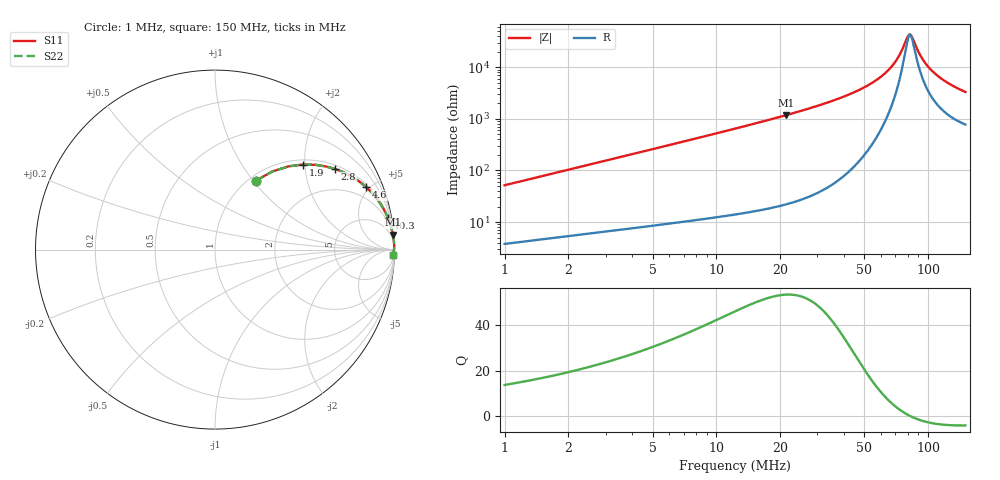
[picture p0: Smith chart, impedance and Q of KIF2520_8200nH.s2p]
!version-2
!date-12.2020
!Series
# MHz S RI R 50
!Freq ReS11 ImS11 ReS21 ImS21 ReS12 ImS12 ReS22 ImS22
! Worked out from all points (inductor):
!   498 points, 1 MHz to 150 MHz, reference 50 ohm
!   read as one part in series: L = 8.2 uH near 1.6 MHz
!   highest Q = 53.6 at 21.4 MHz (marker M1), where L = 8.8 uH
!   self-resonance near 82 MHz
!   S11 on the Smith chart (normalised r, x): 1 MHz: 1.08, +1.03; 1.9 MHz: 1.10, +1.96; 2.8 MHz: 1.13, +2.89; 4.6 MHz: 1.16, +4.75; 10.3 MHz: 1, +11; 150 MHz: 17, -65
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1  0.2269 0.3839  0.7731 -0.3839  0.7731 -0.3839  0.2269 0.3839
1.9  0.4908 0.4741  0.5092 -0.4741  0.5092 -0.4741  0.4908 0.4741
2.8  0.6694 0.4491  0.3306 -0.4491  0.3306 -0.4491  0.6694 0.4491
3.7  0.7765 0.398  0.2235 -0.398  0.2235 -0.398  0.7765 0.398
4.6  0.8415 0.3485  0.1585 -0.3485  0.1585 -0.3485  0.8415 0.3485
6.7  0.9173 0.2616  0.0827 -0.2616  0.0827 -0.2616  0.9173 0.2616
10.3  0.9629 0.1777  0.0371 -0.1777  0.0371 -0.1777  0.9629 0.1777
15.1  0.9825 0.1216  0.0175 -0.1216  0.0175 -0.1216  0.9825 0.1216
21.4  0.9914 0.0836  0.00863 -0.0836  0.00863 -0.0836  0.9914 0.0836
25.9  0.9942 0.067  0.0058 -0.067  0.0058 -0.067  0.9942 0.067
50.8  0.9982 0.0235  0.00176 -0.0235  0.00176 -0.0235  0.9982 0.0235
59.2  0.9983 0.0157  0.00166 -0.0157  0.00166 -0.0157  0.9983 0.0157
65.8  0.9983 0.0105  0.00174 -0.0105  0.00174 -0.0105  0.9983 0.0105
71.2  0.9981 0.00678  0.00188 -0.00678  0.00188 -0.00678  0.9981 0.00678
75.7  0.998 0.00389  0.00203 -0.00389  0.00203 -0.00389  0.998 0.00389
80.2  0.9978 0.00119  0.00222 -0.00119  0.00222 -0.00119  0.9978 0.00119
82.6  0.9977 -0.000182  0.00233 0.000182  0.00233 0.000182  0.9977 -0.000182
91.9  0.9972 -0.00515  0.00283 0.00515  0.00283 0.00515  0.9972 -0.00515
100.6  0.9966 -0.00937  0.00339 0.00937  0.00339 0.00937  0.9966 -0.00937
111.4  0.9958 -0.0142  0.00419 0.0142  0.00419 0.0142  0.9958 -0.0142
125.2  0.9946 -0.0198  0.00535 0.0198  0.00535 0.0198  0.9946 -0.0198
150  0.9922 -0.0288  0.00782 0.0288  0.00782 0.0288  0.9922 -0.0288
